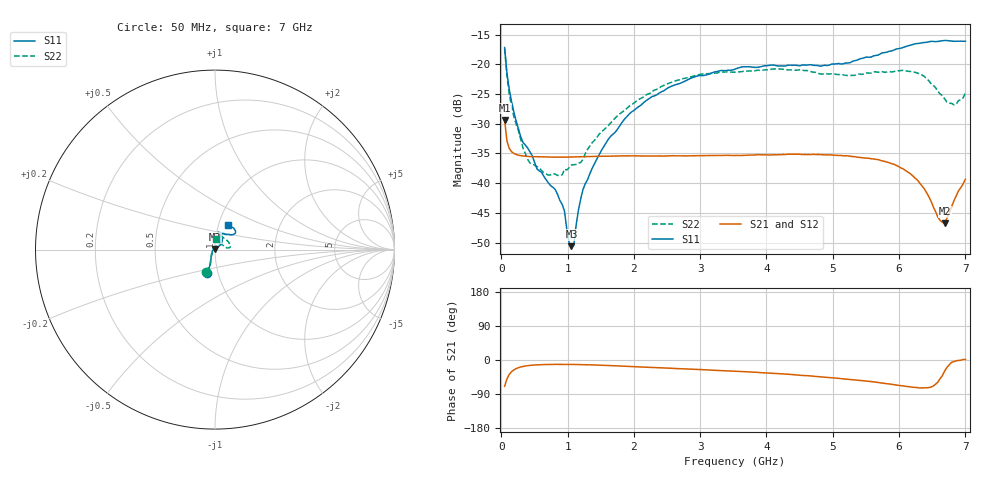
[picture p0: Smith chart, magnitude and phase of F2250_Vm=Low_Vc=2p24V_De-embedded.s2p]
! Integrated Device Technology
! Corporate Headquarters
! 6024 Silver Creek Valley Road
! San Jose, CA 95138  USA
! Phone:  1-408-284-8200
! Toll Free:  1-800-223-1366
! Webpage:  http://www.idt.com/
! Timing and RF Division
! 515 Groton Road, Suite 102
! Westford, MA 01886-6024
! Device:  F2250
! Description: Voltage Variable RF Attenuator
! Frequency:  50.0 -  6000.00 MHz
! Package:  3x3 mm Thin QFN Plastic Package: 16 pin
! Ports:  2 RF, 3 DC
!  Pin  1  = GND
!  Pin  2  = NC
!  Pin  3  = RF1  = Port 1
!  Pin  4  = NC
!  Pin  5  = GND
!  Pin  6  = GND
!  Pin  7  = GND
!  Pin  8  = GND
!  Pin  9  = NC
!  Pin 10  = RF2  = Port 2
!  Pin 11  = NC
!  Pin 12  = GND
!  Pin 13  = GND
!  Pin 14  = VCNTRL
!  Pin 15  = VDD
!  Pin 16  = VMODE
! Vcntrl:  2.240 Volts
! Vmode:  +0.000 Volts
! Vdd:  +3.30  Volts
! Current:  1.178 mA
! Data:  The device was measured on a the F2250 evaluation board which has
!  individual transmission lines to the RF pins.  Data was collected
!  using a calibrated network analyzer.  The evaluation board was
!  de-embedded using a TRL calibration technique.
!  The reference plane is the edge of the package pin.
! Misc:  SN 10
!  Action Tracker AT0258
! Date Measured:  2014-11-26
! Date:  2015-10-15  MJV
! Note:
!  Integrated Device Technology supplies this data as a sample of measured
!  data at the package pin for this product.  Your particular data for this
!  product may vary.
!  Data was taken at 25 degrees C.
!  Integrated Device Technology reserves the right to change this data at anytime.
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# GHz S dB R 50
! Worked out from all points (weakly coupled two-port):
!   201 points, 50 MHz to 7 GHz, reference 50 ohm
!   highest |S21| = -29.39 dB at 50 MHz (marker M1); lowest = -46.7 dB at 6.687 GHz (marker M2)
!   lowest |S11| = -50.6 dB at 1.058 GHz (marker M3), VSWR 1.01, Z = 49.8 + j0.248 ohm
!   |S11| at or under -10 dB: start of sweep to end of sweep
!   |S22| runs from -38.7 to -17.4 dB; largest |S21 - S12| = 6.7e-05
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0.05  -17.18 -108.6  -29.39 -69.6  -29.39 -69.5  -17.36 -110.6
0.08475  -21.44 -107.4  -32.87 -50.1  -32.87 -50.1  -21.88 -109.2
0.15425  -26.24 -116.6  -34.70 -31.0  -34.69 -31.0  -27.06 -120.5
0.29325  -32.19 -127.8  -35.36 -18.4  -35.36 -18.4  -32.63 -134.3
0.3975  -34.09 -141.6  -35.49 -15.0  -35.49 -14.9  -35.98 -157.7
0.71025  -39.95 -168.3  -35.61 -11.8  -35.60 -11.8  -38.65 154.2
0.91875  -43.58 158.2  -35.62 -11.5  -35.62 -11.6  -38.60 128.3
0.9535  -44.70 169.9  -35.62 -11.5  -35.62 -11.5  -37.63 126.4
1.023  -50.04 144.0  -35.60 -11.6  -35.60 -11.6  -37.40 109.7
1.05775  -50.59 122.5  -35.60 -11.7  -35.60 -11.6  -36.95 104.6
1.0925  -50.45 89.6  -35.59 -11.7  -35.59 -11.7  -36.88 99.8
1.162  -44.62 57.0  -35.57 -11.9  -35.57 -11.9  -36.62 88.6
1.2315  -41.09 44.2  -35.55 -12.1  -35.55 -12.2  -36.03 79.0
1.6485  -32.11 41.8  -35.45 -14.7  -35.46 -14.7  -29.88 61.1
2.37825  -24.87 47.3  -35.42 -20.4  -35.42 -20.4  -24.02 55.2
3.525  -20.80 72.5  -35.35 -29.7  -35.35 -29.7  -21.33 74.0
4.7065  -20.17 72.4  -35.15 -42.7  -35.15 -42.7  -21.32 71.8
5.85325  -17.82 40.5  -36.58 -63.4  -36.57 -63.4  -21.24 22.1
6.27025  -16.51 40.1  -39.41 -72.6  -39.41 -72.7  -21.45 8.8
6.68725  -15.99 48.8  -46.72 -28.9  -46.69 -28.4  -25.83 27.7
6.861  -16.12 55.1  -42.15 -2.1  -42.12 -2.1  -26.71 58.0
7  -16.12 63.2  -39.34 1.2  -39.31 1.1  -24.81 83.7
